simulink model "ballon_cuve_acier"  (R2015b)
settings: Solver=ode23t  StartTime=0.0  StopTime=30000  RelTol=1e-3
libraries: fl_lib x6, nesl_utility x4

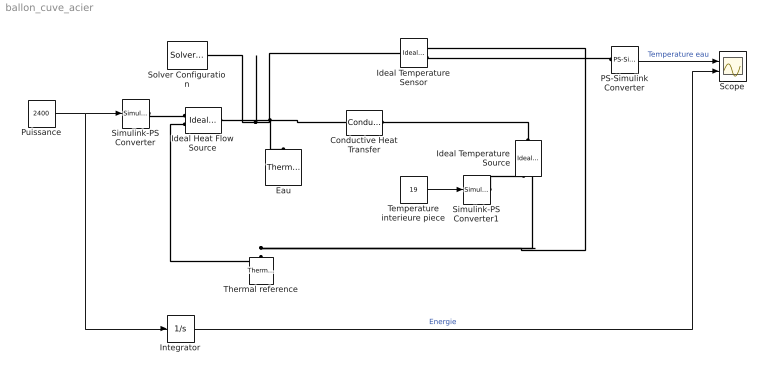
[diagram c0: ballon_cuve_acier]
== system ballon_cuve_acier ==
  Conductive Heat Transfer : fl_lib/Thermal/Thermal Elements/Conductive Heat Transfer  area=2.8 m^2  thickness=2 mm  th_cond=50 W/(m*K)  Q_specify=off  Q_priority=None  Q=0 J/s  T_specify=off  T_priority=None  T=0 K
  Eau : fl_lib/Thermal/Thermal Elements/Thermal Mass  mass=300 kg  sp_heat=4185 J/kg/K  Q_specify=off  Q_priority=None  Q=0 J/s  T_specify=on  T_priority=High  T=15 C
  Ideal Temperature Source : fl_lib/Thermal/Thermal Sources/Ideal Temperature Source
  Ideal Heat Flow Source : fl_lib/Thermal/Thermal Sources/Ideal Heat Flow Source
  Ideal Temperature Sensor : fl_lib/Thermal/Thermal Sensors/Ideal Temperature Sensor
  Integrator : Integrator
  PS-Simulink Converter : nesl_utility/PS-Simulink Converter  PhysicalDomain=network_engine_domain  SubClassName=ps_output  LeftPortType=input  RightPortType=output  PseudoPeriodic=off  Frequencies=[]  Unit=C  AffineConversion=on
  Puissance : Constant  Value=2400
  Scope : Scope  NumInputPorts=2
  Simulink-PS Converter : nesl_utility/Simulink-PS Converter  PhysicalDomain=network_engine_domain  SubClassName=ps_input  LeftPortType=input  RightPortType=output  PseudoPeriodic=off  Frequencies=[]  NoiseDistribution=none  NoiseParameters=[]  Unit=W  AffineConversion=on  InputFiltering=off  SimscapeFilterOrder=1  InputFilterTimeConstant=.001  UdotUserProvided=0
  Simulink-PS Converter1 : nesl_utility/Simulink-PS Converter  PhysicalDomain=network_engine_domain  SubClassName=ps_input  LeftPortType=input  RightPortType=output  PseudoPeriodic=off  Frequencies=[]  NoiseDistribution=none  NoiseParameters=[]  Unit=C  AffineConversion=on  InputFiltering=off  SimscapeFilterOrder=1  InputFilterTimeConstant=.001  UdotUserProvided=1
  Solver Configuration : nesl_utility/Solver Configuration  PhysicalDomain=network_engine_domain  SubClassName=solver  LeftPortType=input  RightPortType=generic  Accelerate=off  Tones=[]  Harmonics=[]  SimulateNoise=off  Profile=off  UseLocalSampling=off  EnableSwitchedLinearOptims=on  FrequencyDomain=off  UseCCode=off  RelTol=0.001  AbsTol=1e-06  MinStep=1e-09  ToWorkspace=off  RevertToSquareIcSolve=off  NumHomotopyIterations=100  PhasorMode=off  PhasorModeNumHarmonics=1  DoDC=off  ResidualTolerance=1e-09  UseLocalSolver=off  LocalSolverChoice=NE_BACKWARD_EULER_ADVANCER  LocalSolverSampleTime=0.001  DoFixedCost=off  MaxNonlinIter=3  MaxModeIter=2  LinearAlgebra=Sparse  DelaysMemoryBudget=1024  AutomaticFiltering=on  FilteringTimeConstant=0.001
  Temperature interieure piece : Constant  Value=19
  Thermal reference : fl_lib/Thermal/Thermal Elements/Thermal Reference
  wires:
  Puissance/1 -> Integrator/1, Simulink-PS Converter/1
  PS-Simulink Converter/1 -> Scope/1  "Temperature eau"
  Integrator/1 -> Scope/2  "Energie"
  Temperature interieure piece/1 -> Simulink-PS Converter1/1
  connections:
  Ideal Heat Flow Source/LConn1 -- Solver Configuration/RConn1 -- Ideal Temperature Sensor/LConn1 -- Conductive Heat Transfer/LConn1 -- Eau/LConn1
  Thermal reference/LConn1 -- Ideal Temperature Source/RConn2 -- Ideal Temperature Sensor/RConn1 -- Ideal Heat Flow Source/RConn2
  Simulink-PS Converter/RConn1 -- Ideal Heat Flow Source/RConn1
  PS-Simulink Converter/LConn1 -- Ideal Temperature Sensor/RConn2
  Simulink-PS Converter1/RConn1 -- Ideal Temperature Source/RConn1
  Ideal Temperature Source/LConn1 -- Conductive Heat Transfer/RConn1
